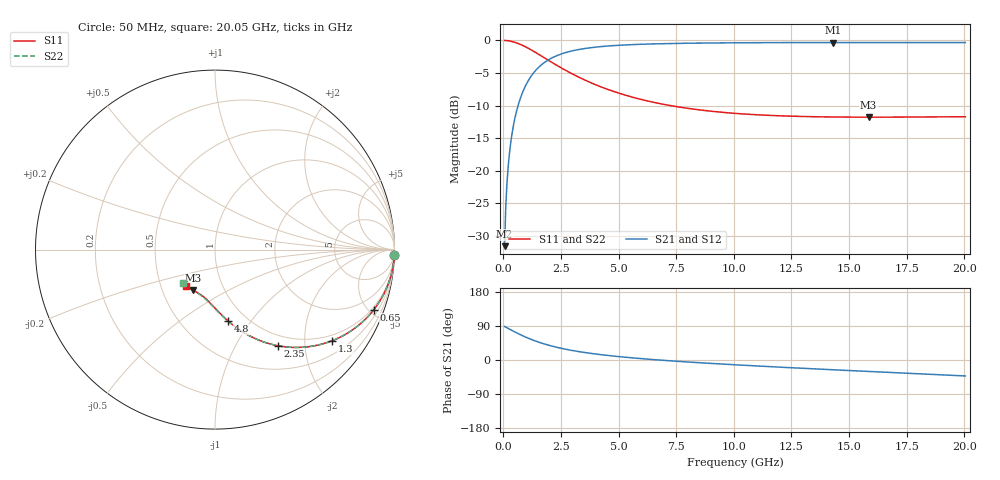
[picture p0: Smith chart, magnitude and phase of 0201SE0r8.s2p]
! AVX Thin Film Operation		Date: August 2001
! Description: Accu-P® Series, Thin Film, SMD, RF Capacitor
! Part Number: 02013J0R8ABW
! 50 MHz  -  20.05 GHz
! Serial Measurements
# mhz S db R 50
!	S11		S21		S12		S22
!	dB	Phase	dB	Phase	dB	Phase	dB	Phase
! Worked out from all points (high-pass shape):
!   401 points, 50 MHz to 20.05 GHz, reference 50 ohm
!   highest |S21| = -0.32 dB at 14.3 GHz (marker M1); lowest = -31.6 dB at 50 MHz (marker M2)
!   |S21| within 3 dB of the highest: 1.804 GHz to end of sweep
!   lowest |S11| = -11.8 dB at 15.85 GHz (marker M3), VSWR 1.69, Z = 35.7 - j17.4 ohm
!   |S11| at or under -10 dB: 7.241 GHz to end of sweep
!   |S22| runs from -11.8 to 0.0 dB; largest |S21 - S12| = 0
!   S11 on the Smith chart (normalised r, x): 50 MHz: 1, -69; 650 MHz: 0.84, -5.35; 1.3 GHz: 0.84, -2.69; 2.35 GHz: 0.83, -1.51; 4.8 GHz: 0.82, -0.78; 20.05 GHz: 0.67, -0.29
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50  -0.00 -1.7  -31.59 88.4  -31.59 88.4  -0.00 -1.7
100  -0.01 -3.3  -25.58 86.7  -25.58 86.7  -0.01 -3.3
200  -0.05 -6.6  -19.60 83.4  -19.60 83.4  -0.05 -6.6
250  -0.07 -8.2  -17.69 81.8  -17.69 81.8  -0.07 -8.2
300  -0.11 -9.8  -16.14 80.2  -16.14 80.2  -0.11 -9.8
450  -0.24 -14.6  -12.75 75.4  -12.75 75.4  -0.24 -14.6
650  -0.48 -20.7  -9.81 69.3  -9.81 69.3  -0.48 -20.7
950  -0.96 -29.2  -7.02 60.8  -7.02 60.8  -0.96 -29.2
1300  -1.65 -37.9  -5.01 52.1  -5.01 52.1  -1.65 -37.9
1750  -2.61 -47.2  -3.46 42.8  -3.46 42.8  -2.61 -47.2
2350  -3.89 -56.9  -2.29 33.0  -2.29 33.0  -3.89 -56.9
2850  -4.88 -63.3  -1.72 26.6  -1.72 26.6  -4.88 -63.3
3400  -5.86 -68.9  -1.31 20.9  -1.31 20.9  -5.86 -69.0
4050  -6.87 -74.4  -1.01 15.4  -1.01 15.4  -6.87 -74.5
4800  -7.85 -79.5  -0.79 10.2  -0.79 10.2  -7.86 -79.7
6750  -9.67 -89.5  -0.51 -0.1  -0.51 -0.1  -9.68 -90.1
10050  -11.20 -101.5  -0.36 -12.6  -0.36 -12.6  -11.21 -103.0
13400  -11.71 -111.3  -0.32 -23.1  -0.32 -23.1  -11.74 -114.0
14300  -11.76 -113.8  -0.32 -25.8  -0.32 -25.8  -11.79 -116.8
15850  -11.79 -117.9  -0.32 -30.2  -0.32 -30.2  -11.82 -121.6
16750  -11.78 -120.3  -0.32 -32.8  -0.32 -32.8  -11.82 -124.4
20050  -11.72 -128.7  -0.33 -42.1  -0.33 -42.1  -11.77 -134.3
